(* Logix 5000 Program export KEP; software revision 30.00; part 8 of 15 *)

ADD_ON_INSTRUCTION Ed25519_VERIFY   (* revision 1.0 20170916, vendor Kenneth A. Fischer *)
// Verifies an Ed25519 Signature.
// Revision note:
// Rev1.0: 20170916 - Initial Release
VAR_IN_OUT
   Temp_C1 : DINT[22]; {required}   // Temp C1 value
   Temp_C2 : DINT[22]; {required}   // Temp C2 value
   Temp_C3 : DINT[22]; {required}   // Temp C3 value
   Temp_C4 : DINT[22]; {required}   // Temp C4 value
   Temp_C5 : DINT[22]; {required}   // Temp C5 value
   Temp_C6 : DINT[22]; {required}   // Temp C6 value
   Temp_C7 : DINT[22]; {required}   // Temp C7 value
   Temp_C8 : DINT[22]; {required}   // Temp C8 value
   Temp_C9 : DINT[22]; {required}   // Temp C9 value
   Temp_C10 : DINT[22]; {required}   // Temp C10 value
   Temp_C11 : DINT[22]; {required}   // Temp C11 value
   Temp_C12 : DINT[22]; {required}   // Temp C12 value
   Temp_D1 : DINT[43]; {required}   // Temp D1 value
   Temp_D2 : DINT[43]; {required}   // Temp D2 value
   Temp_E1 : DINT[32]; {required}   // Temp E1 value
   Temp_E2 : DINT[32]; {required}   // Temp E2 value
   Temp_E3 : DINT[32]; {required}   // Temp E3 value
   Temp_L : LINT[4]; {required}   // Temp L value
   Temp_P1 : POINT; {required}
   Temp_P2 : POINT; {required}
   Temp_P3 : POINT; {required}
   Temp_P4 : POINT; {required}
   Temp_MSG : LINT[1600]; {required}   // Temp MSG holder
   Temp_HASH : LINT[8]; {required}   // Temp HASH value
   Inp_Flags : DINT; {required}
   Inp_PubDH : STRING; {required}
   Inp_Ke : STRING; {required}
   Inp_PubKey : STRING; {required}
   Inp_KsID : LINT; {required}
   Inp_KsPrimeID : LINT; {required}
   Inp_Counter : LINT; {required}
   Inp_Sig_R : STRING; {required}
   Inp_Sig_S : STRING; {required}
END_VAR
VAR_OUTPUT
   Out_Status : INT; {access Read Only, visible}
   SEQCTRL_DN : BOOL; {access Read Only}   // Complete
END_VAR
VAR_INPUT
   SEQCTRL_RESET : BOOL;   // Resets Ed25519 Verify if Toggled True
END_VAR
VAR_OUTPUT
   SEQCTRL_STEP : INT; {access Read Only}
   SEQCTRL_SUBSTEP : INT; {access Read Only}
END_VAR
VAR
   SEQCTRL_CMD : DINT;
   SEQCTRL_CMD_TABLE : DINT[70];
   SEQCTRL_DONE : DINT;
   SEQCTRL_NEXT_STEP : INT;
   TEMP : DINT;
   SHA512_SEQ : SHA512_SEQ;
   SEQCTRL_ONS : DINT;
   B512_HtoD : B512_HtoD;
   B256_MODL1 : B256_MODL;
   POINT_MUL1 : POINT_MUL;
   B256_EtoL : B256_EtoL;
   B256_StoC : B256_StoC;
   B256_CtoE : B256_CtoE;
   POINT_DEC1 : POINT_DEC;
   POINT_DEC2 : POINT_DEC;
   POINT_ADD : POINT_ADD;
   B256_StoC_LE : B256_StoC_LE;
   POINT_MUL2 : POINT_MUL;
   EQUAL : BOOL;
   POINT_ENC1 : POINT_ENC;
   POINT_ENC2 : POINT_ENC;
   Wrk_Out : DINT[2];
END_VAR

ROUTINE Logic   (* ladder *)
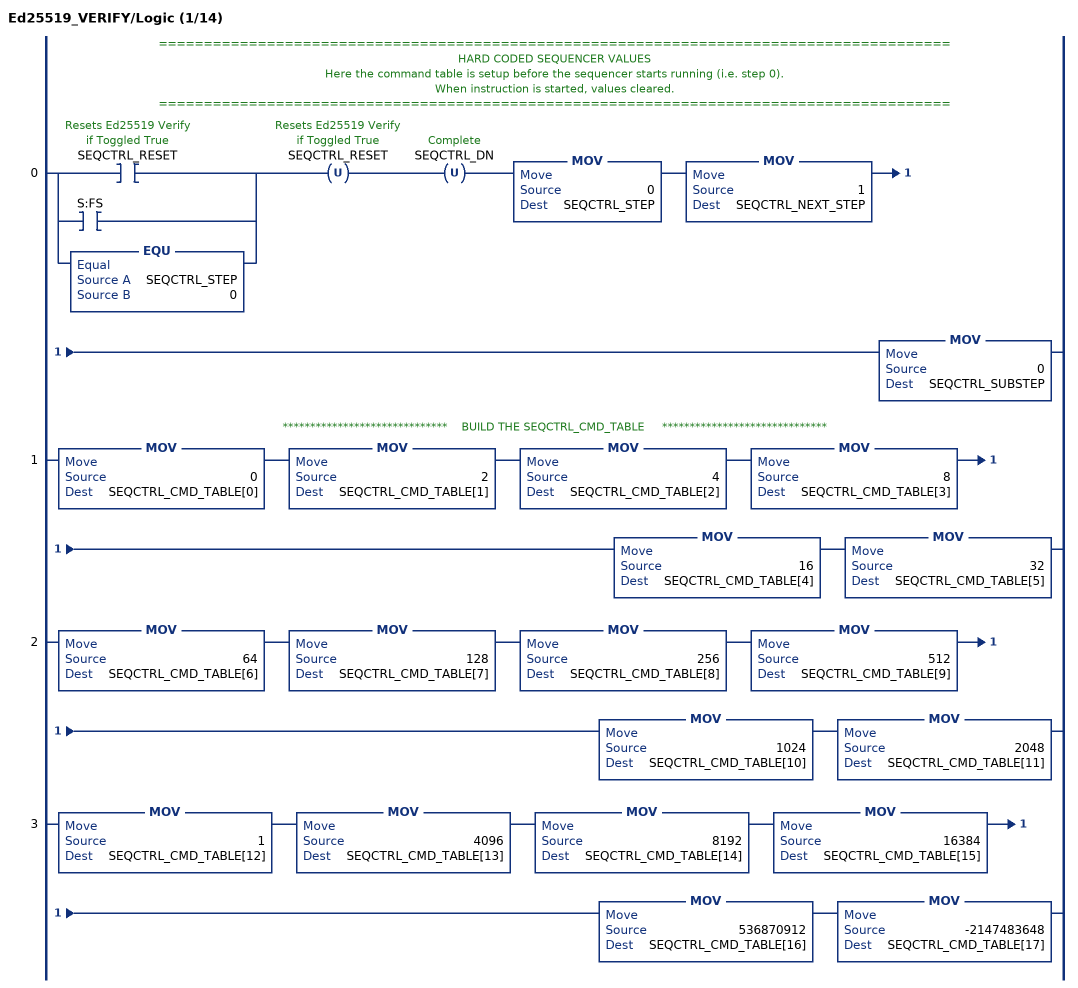
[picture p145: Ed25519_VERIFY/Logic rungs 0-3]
   // ========================================================================================
   // HARD CODED SEQUENCER VALUES
   // Here the command table is setup before the sequencer starts running (i.e. step 0).
   // When instruction is started, values cleared.
   // ========================================================================================
   0: [[XIC(SEQCTRL_RESET) ,XIC(S:FS) ] ,EQU(SEQCTRL_STEP,0) ]OTU(SEQCTRL_RESET)OTU(SEQCTRL_DN)MOV(0,SEQCTRL_STEP)MOV(1,SEQCTRL_NEXT_STEP)MOV(0,SEQCTRL_SUBSTEP);
   // ******************************    BUILD THE SEQCTRL_CMD_TABLE     ******************************
   1: MOV(0,SEQCTRL_CMD_TABLE[0])MOV(2,SEQCTRL_CMD_TABLE[1])MOV(4,SEQCTRL_CMD_TABLE[2])MOV(8,SEQCTRL_CMD_TABLE[3])MOV(16,SEQCTRL_CMD_TABLE[4])MOV(32,SEQCTRL_CMD_TABLE[5]);
   2: MOV(64,SEQCTRL_CMD_TABLE[6])MOV(128,SEQCTRL_CMD_TABLE[7])MOV(256,SEQCTRL_CMD_TABLE[8])MOV(512,SEQCTRL_CMD_TABLE[9])MOV(1024,SEQCTRL_CMD_TABLE[10])MOV(2048,SEQCTRL_CMD_TABLE[11]);
   3: MOV(1,SEQCTRL_CMD_TABLE[12])MOV(4096,SEQCTRL_CMD_TABLE[13])MOV(8192,SEQCTRL_CMD_TABLE[14])MOV(16384,SEQCTRL_CMD_TABLE[15])MOV(536870912,SEQCTRL_CMD_TABLE[16])MOV(-2147483648,SEQCTRL_CMD_TABLE[17]);
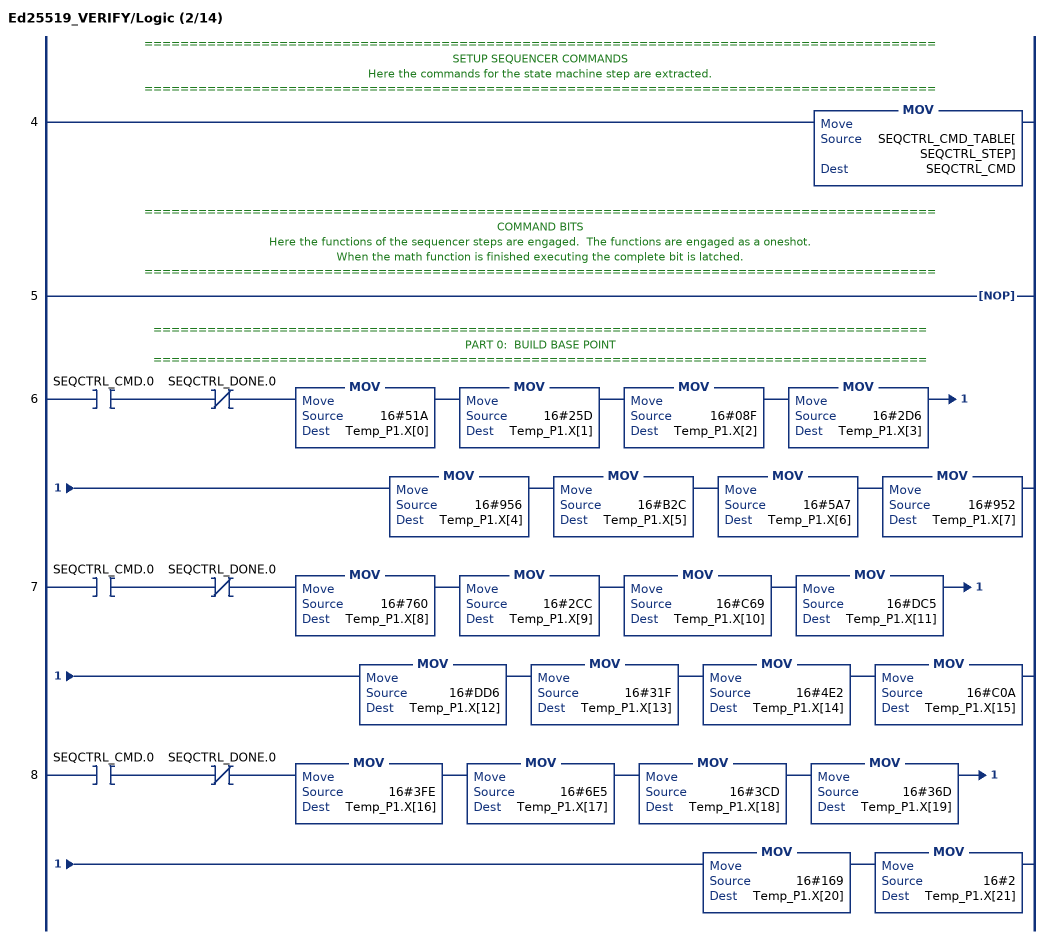
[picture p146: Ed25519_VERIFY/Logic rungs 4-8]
   // ========================================================================================
   // SETUP SEQUENCER COMMANDS
   // Here the commands for the state machine step are extracted.
   // ========================================================================================
   4: MOV(SEQCTRL_CMD_TABLE[SEQCTRL_STEP],SEQCTRL_CMD);
   // ========================================================================================
   // COMMAND BITS
   // Here the functions of the sequencer steps are engaged.  The functions are engaged as a oneshot.
   // When the math function is finished executing the complete bit is latched.
   // ========================================================================================
   5: NOP();
   // ======================================================================================
   // PART 0:  BUILD BASE POINT
   // ======================================================================================
   6: XIC(SEQCTRL_CMD.0)XIO(SEQCTRL_DONE.0)MOV(16#51A,Temp_P1.X[0])MOV(16#25D,Temp_P1.X[1])MOV(16#08F,Temp_P1.X[2])MOV(16#2D6,Temp_P1.X[3])MOV(16#956,Temp_P1.X[4])MOV(16#B2C,Temp_P1.X[5])MOV(16#5A7,Temp_P1.X[6])MOV(16#952,Temp_P1.X[7]);
   7: XIC(SEQCTRL_CMD.0)XIO(SEQCTRL_DONE.0)MOV(16#760,Temp_P1.X[8])MOV(16#2CC,Temp_P1.X[9])MOV(16#C69,Temp_P1.X[10])MOV(16#DC5,Temp_P1.X[11])MOV(16#DD6,Temp_P1.X[12])MOV(16#31F,Temp_P1.X[13])MOV(16#4E2,Temp_P1.X[14])MOV(16#C0A,Temp_P1.X[15]);
   8: XIC(SEQCTRL_CMD.0)XIO(SEQCTRL_DONE.0)MOV(16#3FE,Temp_P1.X[16])MOV(16#6E5,Temp_P1.X[17])MOV(16#3CD,Temp_P1.X[18])MOV(16#36D,Temp_P1.X[19])MOV(16#169,Temp_P1.X[20])MOV(16#2,Temp_P1.X[21]);
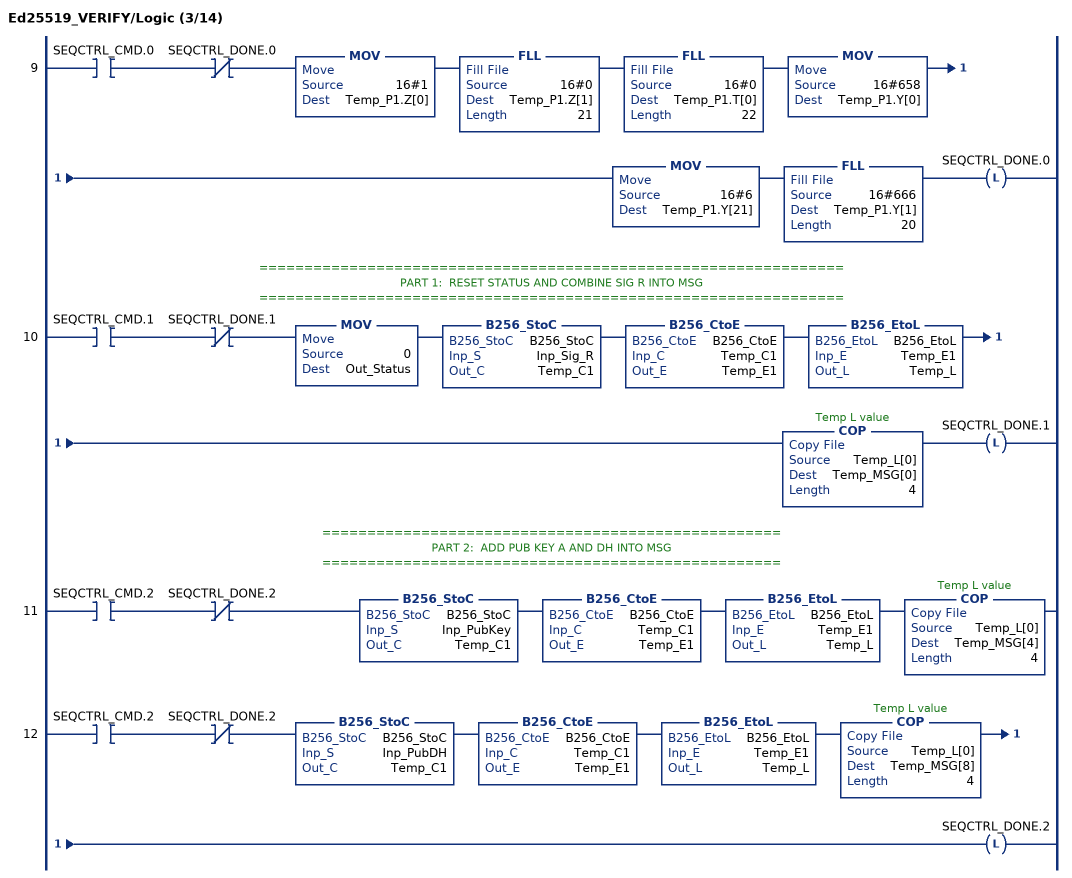
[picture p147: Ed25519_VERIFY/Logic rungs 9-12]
   9: XIC(SEQCTRL_CMD.0)XIO(SEQCTRL_DONE.0)MOV(16#1,Temp_P1.Z[0])FLL(16#0,Temp_P1.Z[1],21)FLL(16#0,Temp_P1.T[0],22)MOV(16#658,Temp_P1.Y[0])MOV(16#6,Temp_P1.Y[21])FLL(16#666,Temp_P1.Y[1],20)OTL(SEQCTRL_DONE.0);
   // =================================================================
   // PART 1:  RESET STATUS AND COMBINE SIG R INTO MSG
   // =================================================================
   10: XIC(SEQCTRL_CMD.1)XIO(SEQCTRL_DONE.1)MOV(0,Out_Status)B256_StoC(B256_StoC,Inp_Sig_R,Temp_C1)B256_CtoE(B256_CtoE,Temp_C1,Temp_E1)B256_EtoL(B256_EtoL,Temp_E1,Temp_L)COP(Temp_L[0],Temp_MSG[0],4)OTL(SEQCTRL_DONE.1);
   // ===================================================
   // PART 2:  ADD PUB KEY A AND DH INTO MSG
   // ===================================================
   11: XIC(SEQCTRL_CMD.2)XIO(SEQCTRL_DONE.2)B256_StoC(B256_StoC,Inp_PubKey,Temp_C1)B256_CtoE(B256_CtoE,Temp_C1,Temp_E1)B256_EtoL(B256_EtoL,Temp_E1,Temp_L)COP(Temp_L[0],Temp_MSG[4],4);
   12: XIC(SEQCTRL_CMD.2)XIO(SEQCTRL_DONE.2)B256_StoC(B256_StoC,Inp_PubDH,Temp_C1)B256_CtoE(B256_CtoE,Temp_C1,Temp_E1)B256_EtoL(B256_EtoL,Temp_E1,Temp_L)COP(Temp_L[0],Temp_MSG[8],4)OTL(SEQCTRL_DONE.2);
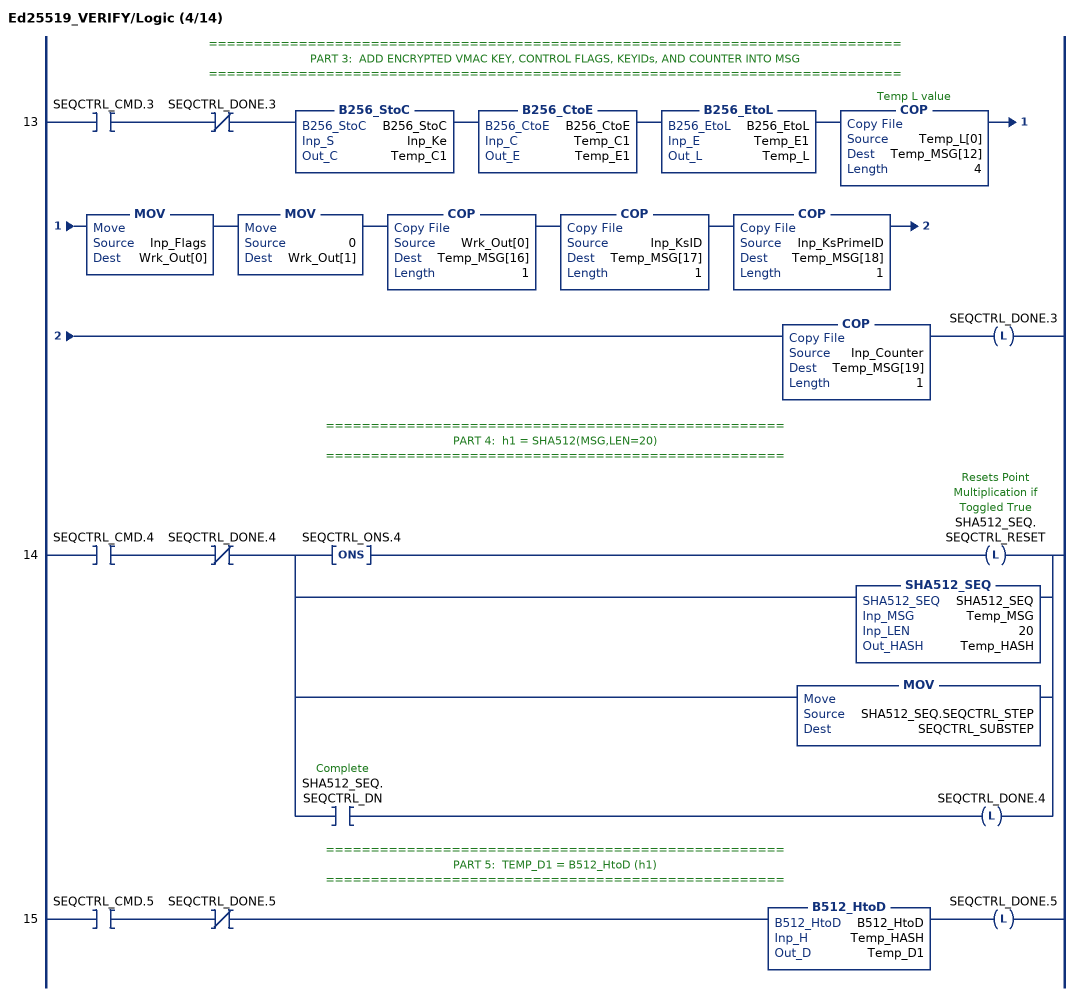
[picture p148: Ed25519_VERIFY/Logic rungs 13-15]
   // =============================================================================
   // PART 3:  ADD ENCRYPTED VMAC KEY, CONTROL FLAGS, KEYIDs, AND COUNTER INTO MSG
   // =============================================================================
   13: XIC(SEQCTRL_CMD.3)XIO(SEQCTRL_DONE.3)B256_StoC(B256_StoC,Inp_Ke,Temp_C1)B256_CtoE(B256_CtoE,Temp_C1,Temp_E1)B256_EtoL(B256_EtoL,Temp_E1,Temp_L)COP(Temp_L[0],Temp_MSG[12],4)MOV(Inp_Flags,Wrk_Out[0])MOV(0,Wrk_Out[1])COP(Wrk_Out[0],Temp_MSG[16],1)COP(Inp_KsID,Temp_MSG[17],1)COP(Inp_KsPrimeID,Temp_MSG[18],1)COP(Inp_Counter,Temp_MSG[19],1)OTL(SEQCTRL_DONE.3);
   // ===================================================
   // PART 4:  h1 = SHA512(MSG,LEN=20)
   // ===================================================
   14: XIC(SEQCTRL_CMD.4)XIO(SEQCTRL_DONE.4)[ONS(SEQCTRL_ONS.4) OTL(SHA512_SEQ.SEQCTRL_RESET) ,SHA512_SEQ(SHA512_SEQ,Temp_MSG,20,Temp_HASH) ,MOV(SHA512_SEQ.SEQCTRL_STEP,SEQCTRL_SUBSTEP) ,XIC(SHA512_SEQ.SEQCTRL_DN) OTL(SEQCTRL_DONE.4) ];
   // ===================================================
   // PART 5:  TEMP_D1 = B512_HtoD (h1)
   // ===================================================
   15: XIC(SEQCTRL_CMD.5)XIO(SEQCTRL_DONE.5)B512_HtoD(B512_HtoD,Temp_HASH,Temp_D1)OTL(SEQCTRL_DONE.5);
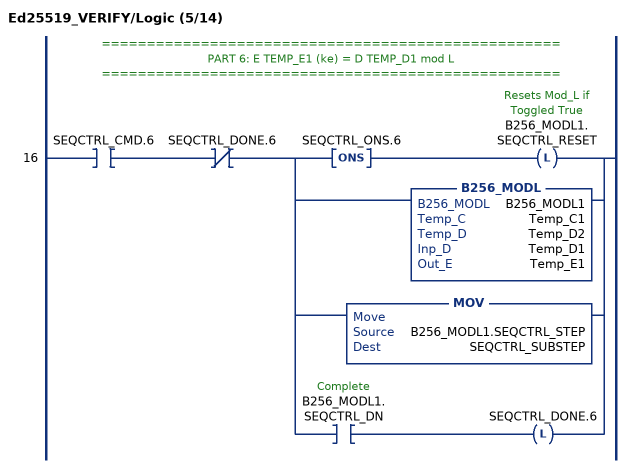
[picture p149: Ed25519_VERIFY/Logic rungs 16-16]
   // ===================================================
   // PART 6: E TEMP_E1 (ke) = D TEMP_D1 mod L
   // ===================================================
   16: XIC(SEQCTRL_CMD.6)XIO(SEQCTRL_DONE.6)[ONS(SEQCTRL_ONS.6) OTL(B256_MODL1.SEQCTRL_RESET) ,B256_MODL(B256_MODL1,Temp_C1,Temp_D2,Temp_D1,Temp_E1) ,MOV(B256_MODL1.SEQCTRL_STEP,SEQCTRL_SUBSTEP) ,XIC(B256_MODL1.SEQCTRL_DN) OTL(SEQCTRL_DONE.6) ];
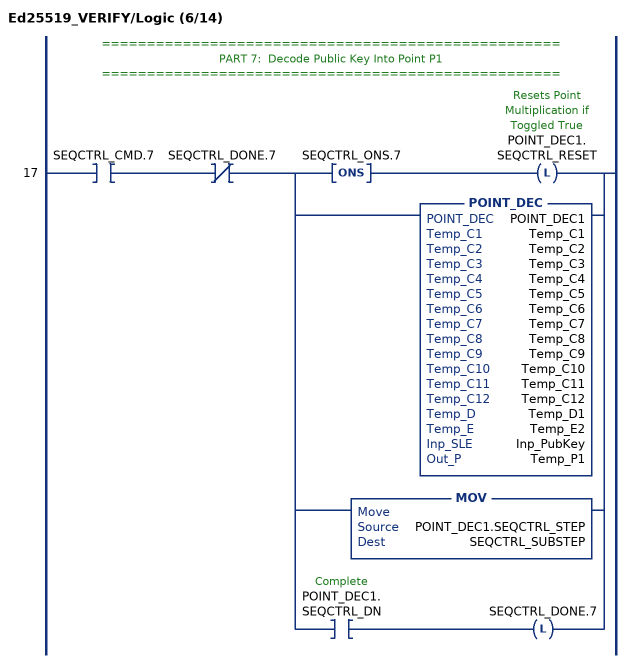
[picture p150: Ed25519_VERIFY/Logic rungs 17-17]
   // ===================================================
   // PART 7:  Decode Public Key Into Point P1
   // ===================================================
   17: XIC(SEQCTRL_CMD.7)XIO(SEQCTRL_DONE.7)[ONS(SEQCTRL_ONS.7) OTL(POINT_DEC1.SEQCTRL_RESET) ,POINT_DEC(POINT_DEC1,Temp_C1,Temp_C2,Temp_C3,Temp_C4,Temp_C5,Temp_C6,Temp_C7,Temp_C8,Temp_C9,Temp_C10,Temp_C11,Temp_C12,Temp_D1,Temp_E2,Inp_PubKey,Temp_P1) ,MOV(POINT_DEC1.SEQCTRL_STEP,SEQCTRL_SUBSTEP) ,XIC(POINT_DEC1.SEQCTRL_DN) OTL(SEQCTRL_DONE.7) ];
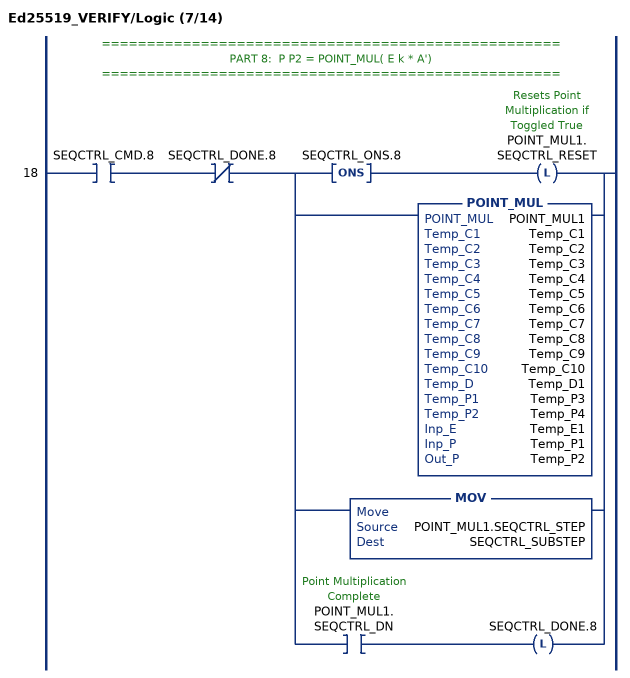
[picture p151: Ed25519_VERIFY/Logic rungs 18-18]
   // ===================================================
   // PART 8:  P P2 = POINT_MUL( E k * A')
   // ===================================================
   18: XIC(SEQCTRL_CMD.8)XIO(SEQCTRL_DONE.8)[ONS(SEQCTRL_ONS.8) OTL(POINT_MUL1.SEQCTRL_RESET) ,POINT_MUL(POINT_MUL1,Temp_C1,Temp_C2,Temp_C3,Temp_C4,Temp_C5,Temp_C6,Temp_C7,Temp_C8,Temp_C9,Temp_C10,Temp_D1,Temp_P3,Temp_P4,Temp_E1,Temp_P1,Temp_P2) ,MOV(POINT_MUL1.SEQCTRL_STEP,SEQCTRL_SUBSTEP) ,XIC(POINT_MUL1.SEQCTRL_DN) OTL(SEQCTRL_DONE.8) ];
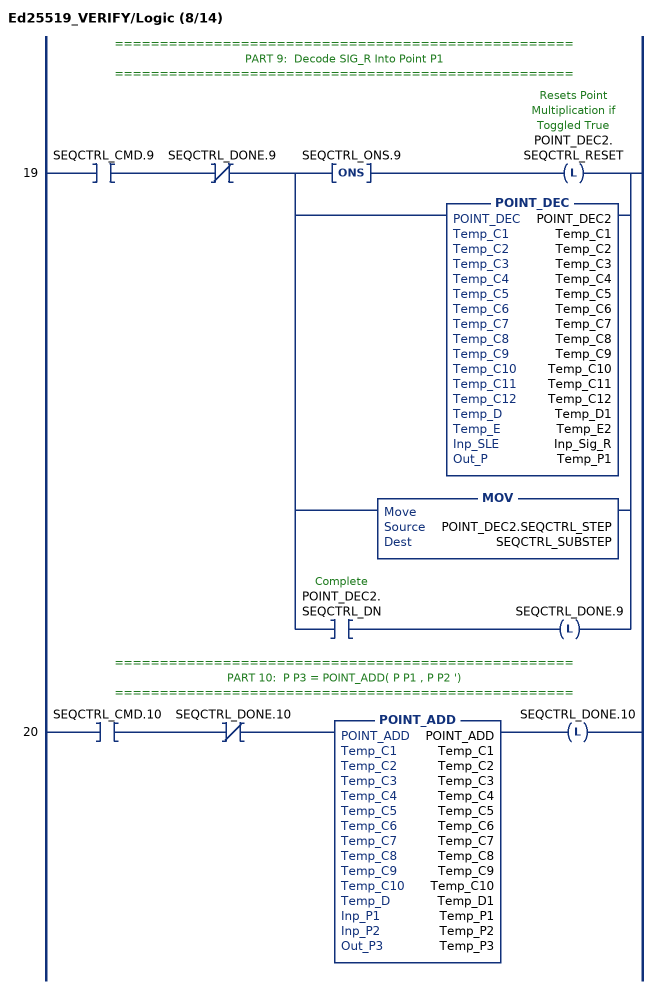
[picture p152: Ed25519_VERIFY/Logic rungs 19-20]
   // ===================================================
   // PART 9:  Decode SIG_R Into Point P1
   // ===================================================
   19: XIC(SEQCTRL_CMD.9)XIO(SEQCTRL_DONE.9)[ONS(SEQCTRL_ONS.9) OTL(POINT_DEC2.SEQCTRL_RESET) ,POINT_DEC(POINT_DEC2,Temp_C1,Temp_C2,Temp_C3,Temp_C4,Temp_C5,Temp_C6,Temp_C7,Temp_C8,Temp_C9,Temp_C10,Temp_C11,Temp_C12,Temp_D1,Temp_E2,Inp_Sig_R,Temp_P1) ,MOV(POINT_DEC2.SEQCTRL_STEP,SEQCTRL_SUBSTEP) ,XIC(POINT_DEC2.SEQCTRL_DN) OTL(SEQCTRL_DONE.9) ];
   // ===================================================
   // PART 10:  P P3 = POINT_ADD( P P1 , P P2 ')
   // ===================================================
   20: XIC(SEQCTRL_CMD.10)XIO(SEQCTRL_DONE.10)POINT_ADD(POINT_ADD,Temp_C1,Temp_C2,Temp_C3,Temp_C4,Temp_C5,Temp_C6,Temp_C7,Temp_C8,Temp_C9,Temp_C10,Temp_D1,Temp_P1,Temp_P2,Temp_P3)OTL(SEQCTRL_DONE.10);
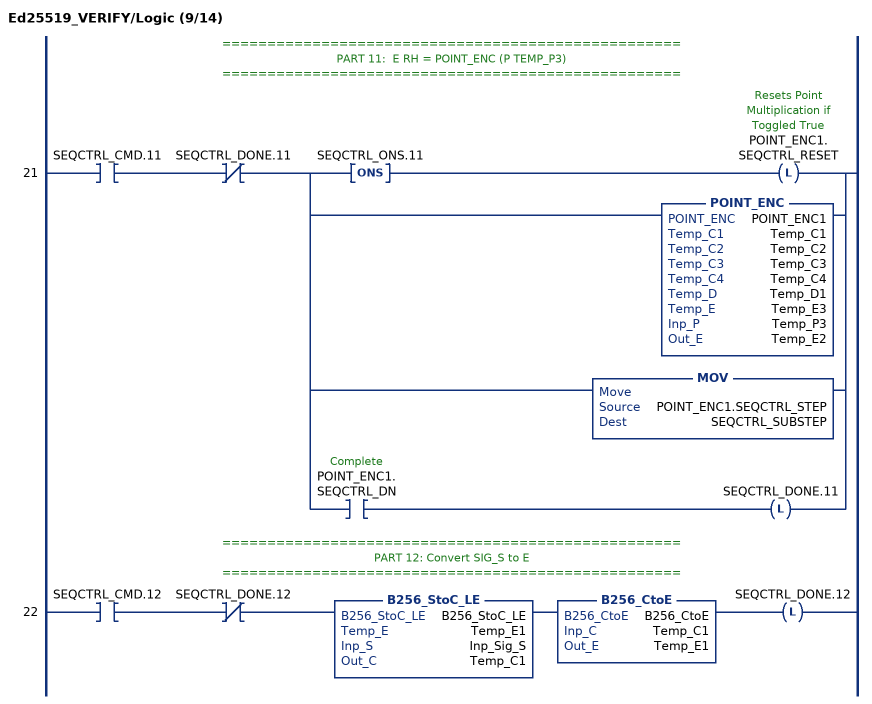
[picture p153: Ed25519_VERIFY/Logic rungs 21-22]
   // ===================================================
   // PART 11:  E RH = POINT_ENC (P TEMP_P3)
   // ===================================================
   21: XIC(SEQCTRL_CMD.11)XIO(SEQCTRL_DONE.11)[ONS(SEQCTRL_ONS.11) OTL(POINT_ENC1.SEQCTRL_RESET) ,POINT_ENC(POINT_ENC1,Temp_C1,Temp_C2,Temp_C3,Temp_C4,Temp_D1,Temp_E3,Temp_P3,Temp_E2) ,MOV(POINT_ENC1.SEQCTRL_STEP,SEQCTRL_SUBSTEP) ,XIC(POINT_ENC1.SEQCTRL_DN) OTL(SEQCTRL_DONE.11) ];
   // ===================================================
   // PART 12: Convert SIG_S to E
   // ===================================================
   22: XIC(SEQCTRL_CMD.12)XIO(SEQCTRL_DONE.12)B256_StoC_LE(B256_StoC_LE,Temp_E1,Inp_Sig_S,Temp_C1)B256_CtoE(B256_CtoE,Temp_C1,Temp_E1)OTL(SEQCTRL_DONE.12);
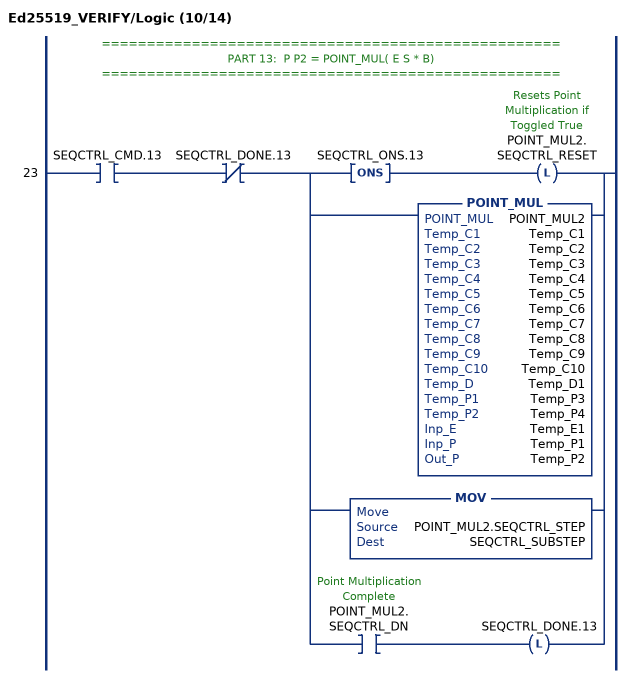
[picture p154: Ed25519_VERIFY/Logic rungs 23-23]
   // ===================================================
   // PART 13:  P P2 = POINT_MUL( E S * B)
   // ===================================================
   23: XIC(SEQCTRL_CMD.13)XIO(SEQCTRL_DONE.13)[ONS(SEQCTRL_ONS.13) OTL(POINT_MUL2.SEQCTRL_RESET) ,POINT_MUL(POINT_MUL2,Temp_C1,Temp_C2,Temp_C3,Temp_C4,Temp_C5,Temp_C6,Temp_C7,Temp_C8,Temp_C9,Temp_C10,Temp_D1,Temp_P3,Temp_P4,Temp_E1,Temp_P1,Temp_P2) ,MOV(POINT_MUL2.SEQCTRL_STEP,SEQCTRL_SUBSTEP) ,XIC(POINT_MUL2.SEQCTRL_DN) OTL(SEQCTRL_DONE.13) ];
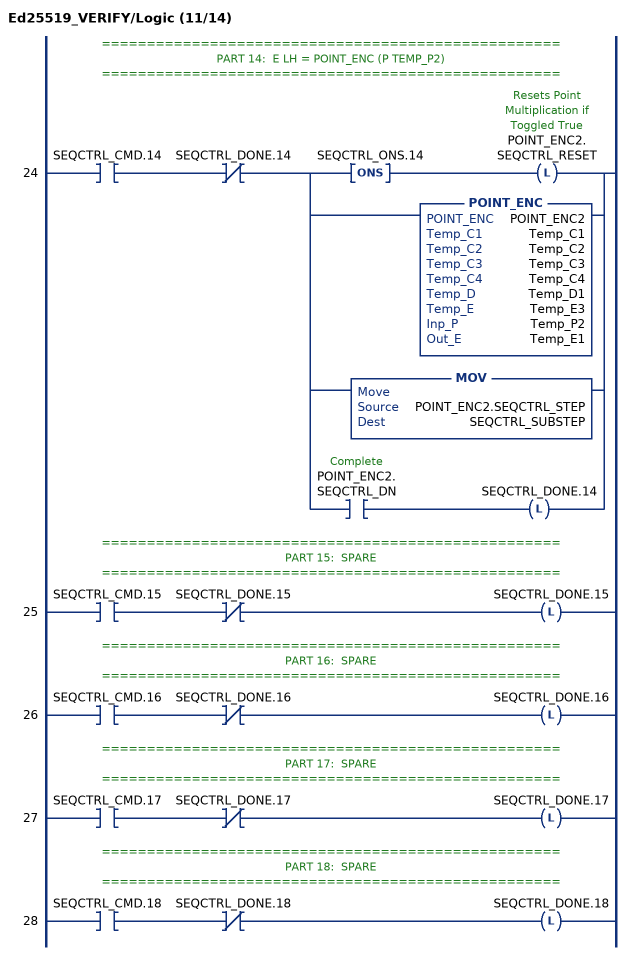
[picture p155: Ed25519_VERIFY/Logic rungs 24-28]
   // ===================================================
   // PART 14:  E LH = POINT_ENC (P TEMP_P2)
   // ===================================================
   24: XIC(SEQCTRL_CMD.14)XIO(SEQCTRL_DONE.14)[ONS(SEQCTRL_ONS.14) OTL(POINT_ENC2.SEQCTRL_RESET) ,POINT_ENC(POINT_ENC2,Temp_C1,Temp_C2,Temp_C3,Temp_C4,Temp_D1,Temp_E3,Temp_P2,Temp_E1) ,MOV(POINT_ENC2.SEQCTRL_STEP,SEQCTRL_SUBSTEP) ,XIC(POINT_ENC2.SEQCTRL_DN) OTL(SEQCTRL_DONE.14) ];
   // ===================================================
   // PART 15:  SPARE
   // ===================================================
   25: XIC(SEQCTRL_CMD.15)XIO(SEQCTRL_DONE.15)OTL(SEQCTRL_DONE.15);
   // ===================================================
   // PART 16:  SPARE
   // ===================================================
   26: XIC(SEQCTRL_CMD.16)XIO(SEQCTRL_DONE.16)OTL(SEQCTRL_DONE.16);
   // ===================================================
   // PART 17:  SPARE
   // ===================================================
   27: XIC(SEQCTRL_CMD.17)XIO(SEQCTRL_DONE.17)OTL(SEQCTRL_DONE.17);
   // ===================================================
   // PART 18:  SPARE
   // ===================================================
   28: XIC(SEQCTRL_CMD.18)XIO(SEQCTRL_DONE.18)OTL(SEQCTRL_DONE.18);
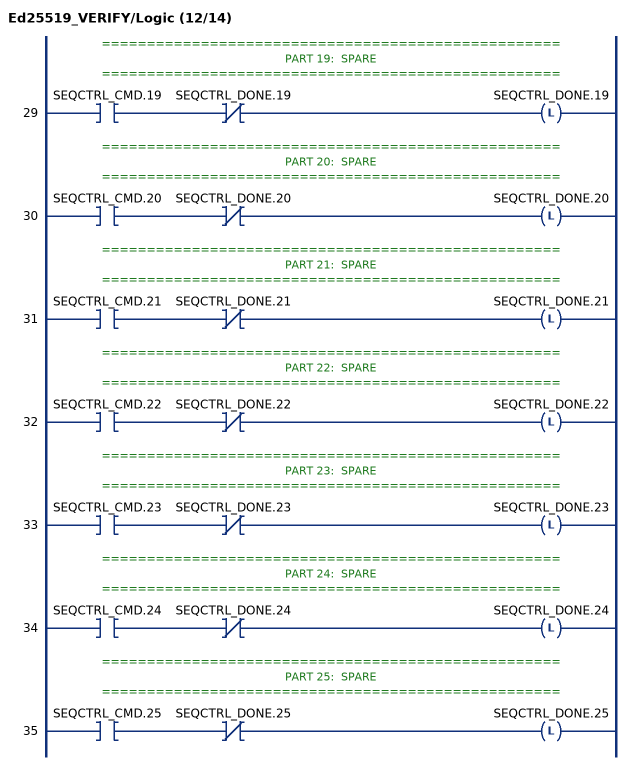
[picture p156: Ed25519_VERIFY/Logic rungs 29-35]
   // ===================================================
   // PART 19:  SPARE
   // ===================================================
   29: XIC(SEQCTRL_CMD.19)XIO(SEQCTRL_DONE.19)OTL(SEQCTRL_DONE.19);
   // ===================================================
   // PART 20:  SPARE
   // ===================================================
   30: XIC(SEQCTRL_CMD.20)XIO(SEQCTRL_DONE.20)OTL(SEQCTRL_DONE.20);
   // ===================================================
   // PART 21:  SPARE
   // ===================================================
   31: XIC(SEQCTRL_CMD.21)XIO(SEQCTRL_DONE.21)OTL(SEQCTRL_DONE.21);
   // ===================================================
   // PART 22:  SPARE
   // ===================================================
   32: XIC(SEQCTRL_CMD.22)XIO(SEQCTRL_DONE.22)OTL(SEQCTRL_DONE.22);
   // ===================================================
   // PART 23:  SPARE
   // ===================================================
   33: XIC(SEQCTRL_CMD.23)XIO(SEQCTRL_DONE.23)OTL(SEQCTRL_DONE.23);
   // ===================================================
   // PART 24:  SPARE
   // ===================================================
   34: XIC(SEQCTRL_CMD.24)XIO(SEQCTRL_DONE.24)OTL(SEQCTRL_DONE.24);
   // ===================================================
   // PART 25:  SPARE
   // ===================================================
   35: XIC(SEQCTRL_CMD.25)XIO(SEQCTRL_DONE.25)OTL(SEQCTRL_DONE.25);
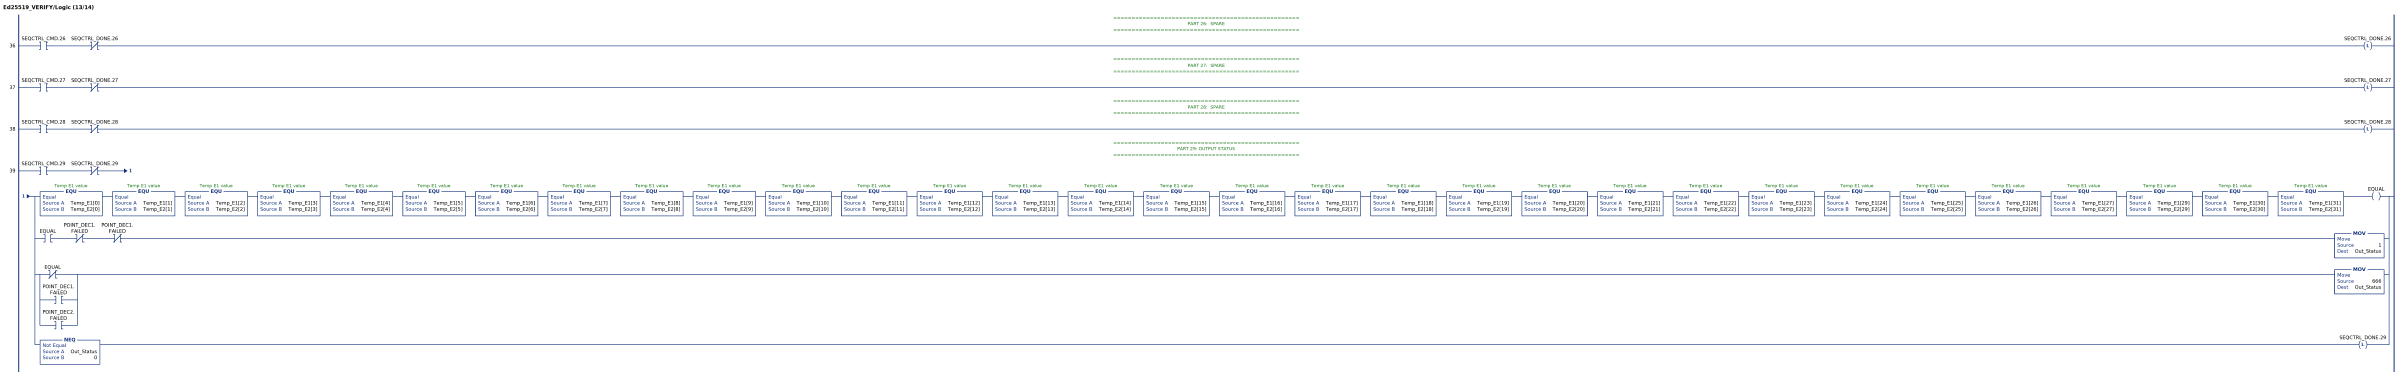
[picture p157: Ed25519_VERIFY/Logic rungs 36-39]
   // ===================================================
   // PART 26:  SPARE
   // ===================================================
   36: XIC(SEQCTRL_CMD.26)XIO(SEQCTRL_DONE.26)OTL(SEQCTRL_DONE.26);
   // ===================================================
   // PART 27:  SPARE
   // ===================================================
   37: XIC(SEQCTRL_CMD.27)XIO(SEQCTRL_DONE.27)OTL(SEQCTRL_DONE.27);
   // ===================================================
   // PART 28:  SPARE
   // ===================================================
   38: XIC(SEQCTRL_CMD.28)XIO(SEQCTRL_DONE.28)OTL(SEQCTRL_DONE.28);
   // ===================================================
   // PART 29: OUTPUT STATUS
   // ===================================================
   39: XIC(SEQCTRL_CMD.29)XIO(SEQCTRL_DONE.29)[EQU(Temp_E1[0],Temp_E2[0]) EQU(Temp_E1[1],Temp_E2[1]) EQU(Temp_E1[2],Temp_E2[2]) EQU(Temp_E1[3],Temp_E2[3]) EQU(Temp_E1[4],Temp_E2[4]) EQU(Temp_E1[5],Temp_E2[5]) EQU(Temp_E1[6],Temp_E2[6]) EQU(Temp_E1[7],Temp_E2[7]) EQU(Temp_E1[8],Temp_E2[8]) EQU(Temp_E1[9],Temp_E2[9]) EQU(Temp_E1[10],Temp_E2[10]) EQU(Temp_E1[11],Temp_E2[11]) EQU(Temp_E1[12],Temp_E2[12]) EQU(Temp_E1[13],Temp_E2[13]) EQU(Temp_E1[14],Temp_E2[14]) EQU(Temp_E1[15],Temp_E2[15]) EQU(Temp_E1[16],Temp_E2[16]) EQU(Temp_E1[17],Temp_E2[17]) EQU(Temp_E1[18],Temp_E2[18]) EQU(Temp_E1[19],Temp_E2[19]) EQU(Temp_E1[20],Temp_E2[20]) EQU(Temp_E1[21],Temp_E2[21]) EQU(Temp_E1[22],Temp_E2[22]) EQU(Temp_E1[23],Temp_E2[23]) EQU(Temp_E1[24],Temp_E2[24]) EQU(Temp_E1[25],Temp_E2[25]) EQU(Temp_E1[26],Temp_E2[26]) EQU(Temp_E1[27],Temp_E2[27]) EQU(Temp_E1[29],Temp_E2[29]) EQU(Temp_E1[30],Temp_E2[30]) EQU(Temp_E1[31],Temp_E2[31]) OTE(EQUAL) ,XIC(EQUAL) XIO(POINT_DEC1.FAILED) XIO(POINT_DEC1.FAILED) MOV(1,Out_Status) ,[XIO(EQUAL) ,XIC(POINT_DEC1.FAILED) ,XIC(POINT_DEC2.FAILED) ] MOV(666,Out_Status) ,NEQ(Out_Status,0) OTL(SEQCTRL_DONE.29) ];
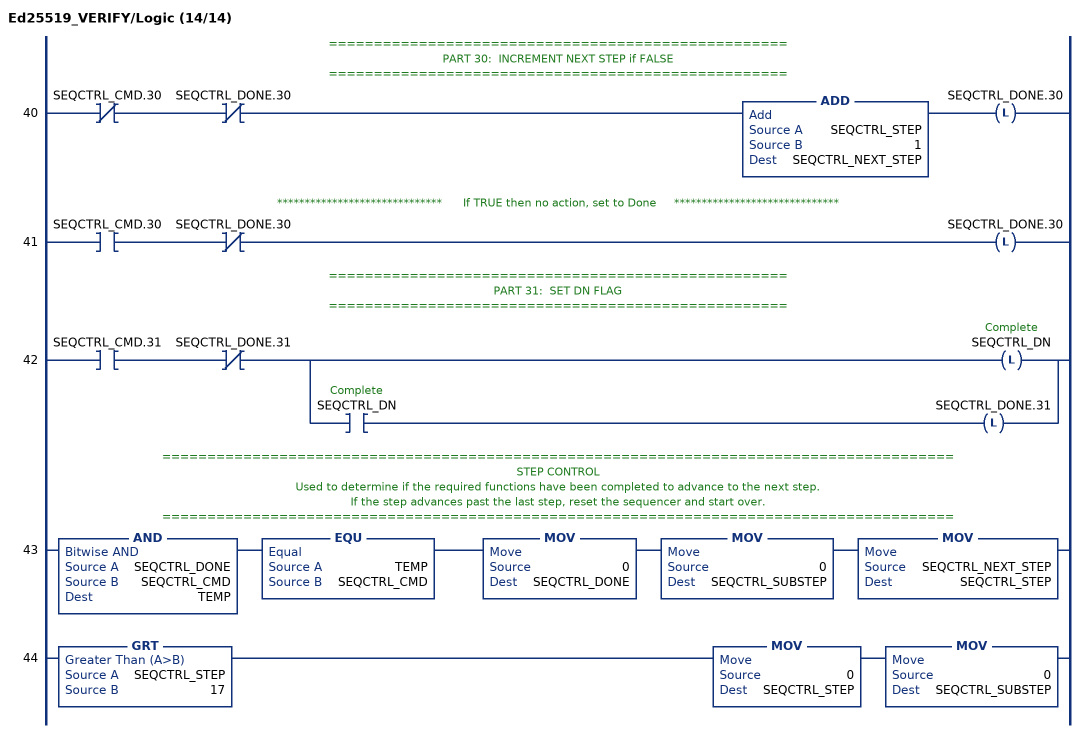
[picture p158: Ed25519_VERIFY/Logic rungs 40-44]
   // ===================================================
   // PART 30:  INCREMENT NEXT STEP if FALSE
   // ===================================================
   40: XIO(SEQCTRL_CMD.30)XIO(SEQCTRL_DONE.30)ADD(SEQCTRL_STEP,1,SEQCTRL_NEXT_STEP)OTL(SEQCTRL_DONE.30);
   // ******************************      If TRUE then no action, set to Done     ******************************
   41: XIC(SEQCTRL_CMD.30)XIO(SEQCTRL_DONE.30)OTL(SEQCTRL_DONE.30);
   // ===================================================
   // PART 31:  SET DN FLAG
   // ===================================================
   42: XIC(SEQCTRL_CMD.31)XIO(SEQCTRL_DONE.31)[OTL(SEQCTRL_DN) ,XIC(SEQCTRL_DN) OTL(SEQCTRL_DONE.31) ];
   // ========================================================================================
   // STEP CONTROL
   // Used to determine if the required functions have been completed to advance to the next step.
   // If the step advances past the last step, reset the sequencer and start over.
   // ========================================================================================
   43: AND(SEQCTRL_DONE,SEQCTRL_CMD,TEMP)EQU(TEMP,SEQCTRL_CMD)MOV(0,SEQCTRL_DONE)MOV(0,SEQCTRL_SUBSTEP)MOV(SEQCTRL_NEXT_STEP,SEQCTRL_STEP);
   44: GRT(SEQCTRL_STEP,17)MOV(0,SEQCTRL_STEP)MOV(0,SEQCTRL_SUBSTEP);
END_ROUTINE
END_ADD_ON_INSTRUCTION

ADD_ON_INSTRUCTION PRNG   (* revision 1.0 20170916, vendor Kenneth A. Fischer *)
// Pseudo-Random Number Generator
// (not proven secure)
// Revision note:
// Rev1.0: 20170916 - Initial Release
VAR_IN_OUT
   Temp_C : DINT[22]; {required}
   Temp_D : DINT[43]; {required}
   Temp_E : DINT[32]; {required}
   Temp_L : LINT[4]; {required}
   Temp_MSG : LINT[1600]; {required}   // Temp MSG holder
   Temp_HASH : LINT[8]; {required}   // Temp HASH value
   Inp_Constant : STRING; {required}
   Inp_Seed : LINT[13]; {required}
   Inp_Counter : LINT; {required}
   Out_PRN : STRING; {required}
END_VAR
VAR_OUTPUT
   SEQCTRL_DN : BOOL; {access Read Only}   // Complete
END_VAR
VAR_INPUT
   SEQCTRL_RESET : BOOL;   // Resets Ed25519 Verify if Toggled True
END_VAR
VAR_OUTPUT
   SEQCTRL_STEP : INT; {access Read Only}
   SEQCTRL_SUBSTEP : INT; {access Read Only}
END_VAR
VAR
   SEQCTRL_CMD : DINT;
   SEQCTRL_CMD_TABLE : DINT[70];
   SEQCTRL_DONE : DINT;
   SEQCTRL_NEXT_STEP : INT;
   TEMP : DINT;
   SHA512_SEQ : SHA512_SEQ;
   SEQCTRL_ONS : DINT;
   Wrk_Out : DINT[2];
   L_INC : L_INC;
   B256_StoC : B256_StoC;
   B256_CtoE : B256_CtoE;
   B256_EtoL : B256_EtoL;
   B512_HtoD : B512_HtoD;
   B256_CtoS : B256_CtoS;
   L_ROTR : L_ROTR;
   L_ADD : L_ADD;
   SwapLint : LINT;
END_VAR

ROUTINE Logic   (* ladder *)
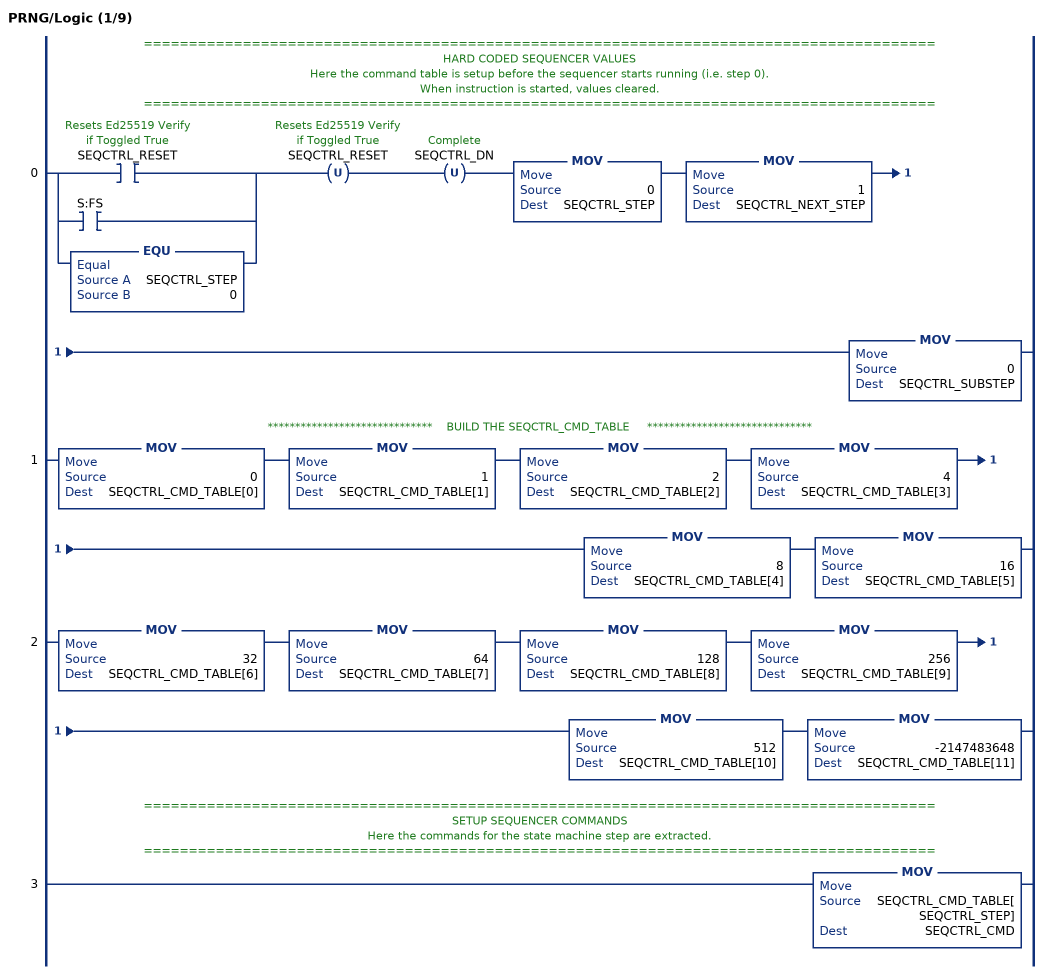
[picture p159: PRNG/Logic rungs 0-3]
   // ========================================================================================
   // HARD CODED SEQUENCER VALUES
   // Here the command table is setup before the sequencer starts running (i.e. step 0).
   // When instruction is started, values cleared.
   // ========================================================================================
   0: [[XIC(SEQCTRL_RESET) ,XIC(S:FS) ] ,EQU(SEQCTRL_STEP,0) ]OTU(SEQCTRL_RESET)OTU(SEQCTRL_DN)MOV(0,SEQCTRL_STEP)MOV(1,SEQCTRL_NEXT_STEP)MOV(0,SEQCTRL_SUBSTEP);
   // ******************************    BUILD THE SEQCTRL_CMD_TABLE     ******************************
   1: MOV(0,SEQCTRL_CMD_TABLE[0])MOV(1,SEQCTRL_CMD_TABLE[1])MOV(2,SEQCTRL_CMD_TABLE[2])MOV(4,SEQCTRL_CMD_TABLE[3])MOV(8,SEQCTRL_CMD_TABLE[4])MOV(16,SEQCTRL_CMD_TABLE[5]);
   2: MOV(32,SEQCTRL_CMD_TABLE[6])MOV(64,SEQCTRL_CMD_TABLE[7])MOV(128,SEQCTRL_CMD_TABLE[8])MOV(256,SEQCTRL_CMD_TABLE[9])MOV(512,SEQCTRL_CMD_TABLE[10])MOV(-2147483648,SEQCTRL_CMD_TABLE[11]);
   // ========================================================================================
   // SETUP SEQUENCER COMMANDS
   // Here the commands for the state machine step are extracted.
   // ========================================================================================
   3: MOV(SEQCTRL_CMD_TABLE[SEQCTRL_STEP],SEQCTRL_CMD);
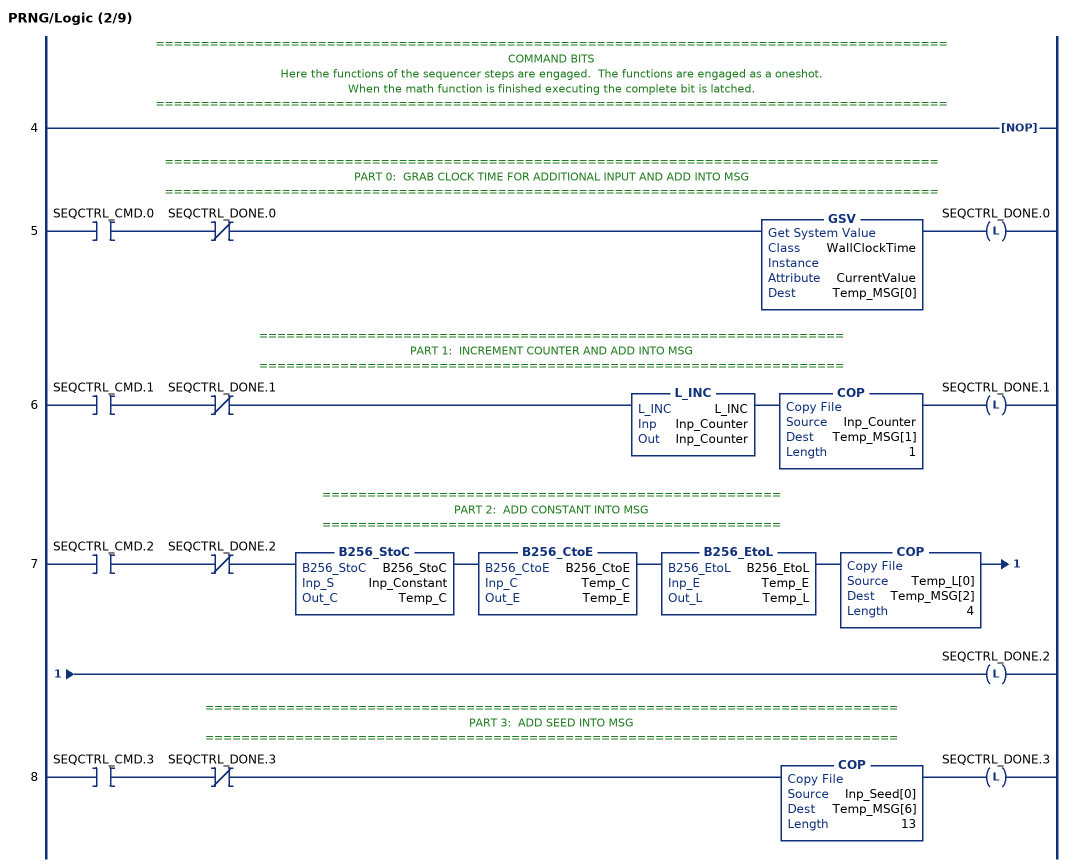
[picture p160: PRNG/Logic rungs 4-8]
   // ========================================================================================
   // COMMAND BITS
   // Here the functions of the sequencer steps are engaged.  The functions are engaged as a oneshot.
   // When the math function is finished executing the complete bit is latched.
   // ========================================================================================
   4: NOP();
   // ======================================================================================
   // PART 0:  GRAB CLOCK TIME FOR ADDITIONAL INPUT AND ADD INTO MSG
   // ======================================================================================
   5: XIC(SEQCTRL_CMD.0)XIO(SEQCTRL_DONE.0)GSV(WallClockTime,,CurrentValue,Temp_MSG[0])OTL(SEQCTRL_DONE.0);
   // =================================================================
   // PART 1:  INCREMENT COUNTER AND ADD INTO MSG
   // =================================================================
   6: XIC(SEQCTRL_CMD.1)XIO(SEQCTRL_DONE.1)L_INC(L_INC,Inp_Counter,Inp_Counter)COP(Inp_Counter,Temp_MSG[1],1)OTL(SEQCTRL_DONE.1);
   // ===================================================
   // PART 2:  ADD CONSTANT INTO MSG
   // ===================================================
   7: XIC(SEQCTRL_CMD.2)XIO(SEQCTRL_DONE.2)B256_StoC(B256_StoC,Inp_Constant,Temp_C)B256_CtoE(B256_CtoE,Temp_C,Temp_E)B256_EtoL(B256_EtoL,Temp_E,Temp_L)COP(Temp_L[0],Temp_MSG[2],4)OTL(SEQCTRL_DONE.2);
   // =============================================================================
   // PART 3:  ADD SEED INTO MSG
   // =============================================================================
   8: XIC(SEQCTRL_CMD.3)XIO(SEQCTRL_DONE.3)COP(Inp_Seed[0],Temp_MSG[6],13)OTL(SEQCTRL_DONE.3);
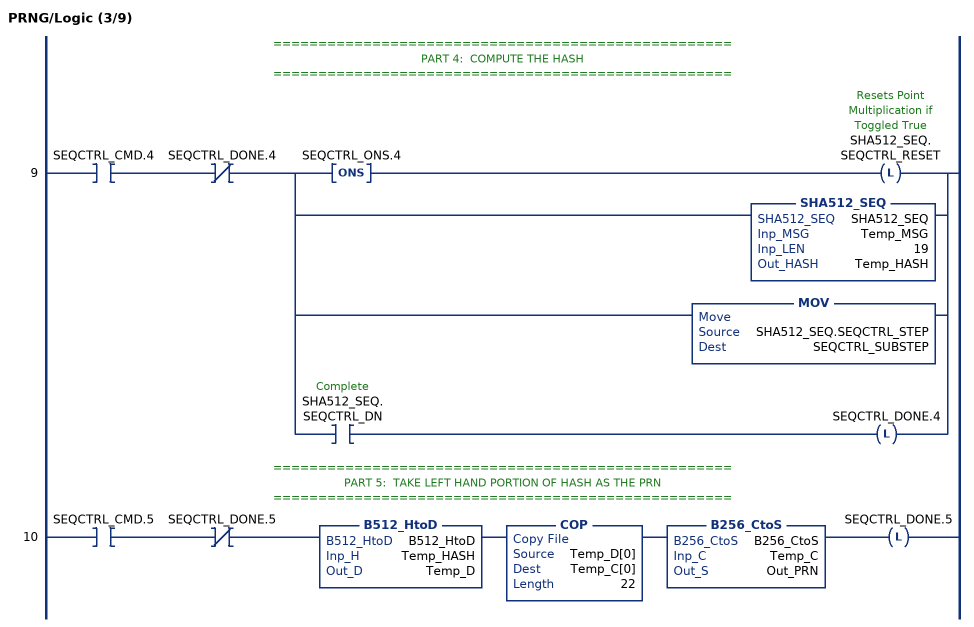
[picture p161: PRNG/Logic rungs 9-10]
   // ===================================================
   // PART 4:  COMPUTE THE HASH
   // ===================================================
   9: XIC(SEQCTRL_CMD.4)XIO(SEQCTRL_DONE.4)[ONS(SEQCTRL_ONS.4) OTL(SHA512_SEQ.SEQCTRL_RESET) ,SHA512_SEQ(SHA512_SEQ,Temp_MSG,19,Temp_HASH) ,MOV(SHA512_SEQ.SEQCTRL_STEP,SEQCTRL_SUBSTEP) ,XIC(SHA512_SEQ.SEQCTRL_DN) OTL(SEQCTRL_DONE.4) ];
   // ===================================================
   // PART 5:  TAKE LEFT HAND PORTION OF HASH AS THE PRN
   // ===================================================
   10: XIC(SEQCTRL_CMD.5)XIO(SEQCTRL_DONE.5)B512_HtoD(B512_HtoD,Temp_HASH,Temp_D)COP(Temp_D[0],Temp_C[0],22)B256_CtoS(B256_CtoS,Temp_C,Out_PRN)OTL(SEQCTRL_DONE.5);
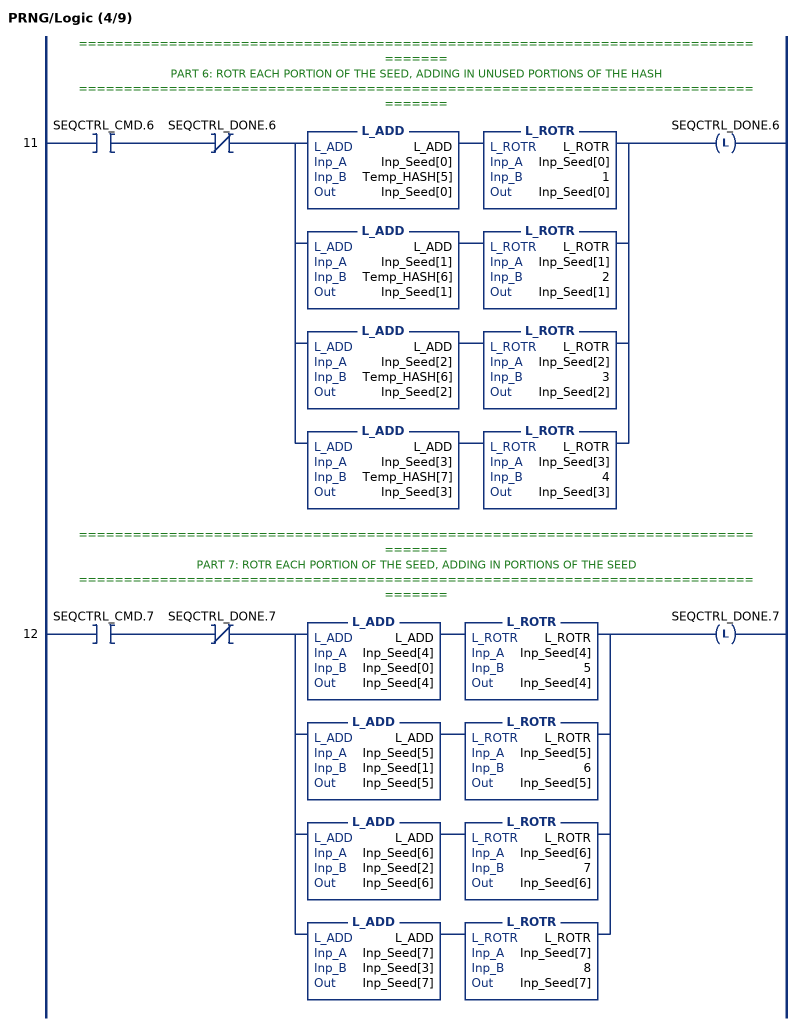
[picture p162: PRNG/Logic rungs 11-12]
   // ==================================================================================
   // PART 6: ROTR EACH PORTION OF THE SEED, ADDING IN UNUSED PORTIONS OF THE HASH
   // ==================================================================================
   11: XIC(SEQCTRL_CMD.6)XIO(SEQCTRL_DONE.6)[L_ADD(L_ADD,Inp_Seed[0],Temp_HASH[5],Inp_Seed[0]) L_ROTR(L_ROTR,Inp_Seed[0],1,Inp_Seed[0]) ,L_ADD(L_ADD,Inp_Seed[1],Temp_HASH[6],Inp_Seed[1]) L_ROTR(L_ROTR,Inp_Seed[1],2,Inp_Seed[1]) ,L_ADD(L_ADD,Inp_Seed[2],Temp_HASH[6],Inp_Seed[2]) L_ROTR(L_ROTR,Inp_Seed[2],3,Inp_Seed[2]) ,L_ADD(L_ADD,Inp_Seed[3],Temp_HASH[7],Inp_Seed[3]) L_ROTR(L_ROTR,Inp_Seed[3],4,Inp_Seed[3]) ]OTL(SEQCTRL_DONE.6);
   // ==================================================================================
   // PART 7: ROTR EACH PORTION OF THE SEED, ADDING IN PORTIONS OF THE SEED
   // ==================================================================================
   12: XIC(SEQCTRL_CMD.7)XIO(SEQCTRL_DONE.7)[L_ADD(L_ADD,Inp_Seed[4],Inp_Seed[0],Inp_Seed[4]) L_ROTR(L_ROTR,Inp_Seed[4],5,Inp_Seed[4]) ,L_ADD(L_ADD,Inp_Seed[5],Inp_Seed[1],Inp_Seed[5]) L_ROTR(L_ROTR,Inp_Seed[5],6,Inp_Seed[5]) ,L_ADD(L_ADD,Inp_Seed[6],Inp_Seed[2],Inp_Seed[6]) L_ROTR(L_ROTR,Inp_Seed[6],7,Inp_Seed[6]) ,L_ADD(L_ADD,Inp_Seed[7],Inp_Seed[3],Inp_Seed[7]) L_ROTR(L_ROTR,Inp_Seed[7],8,Inp_Seed[7]) ]OTL(SEQCTRL_DONE.7);
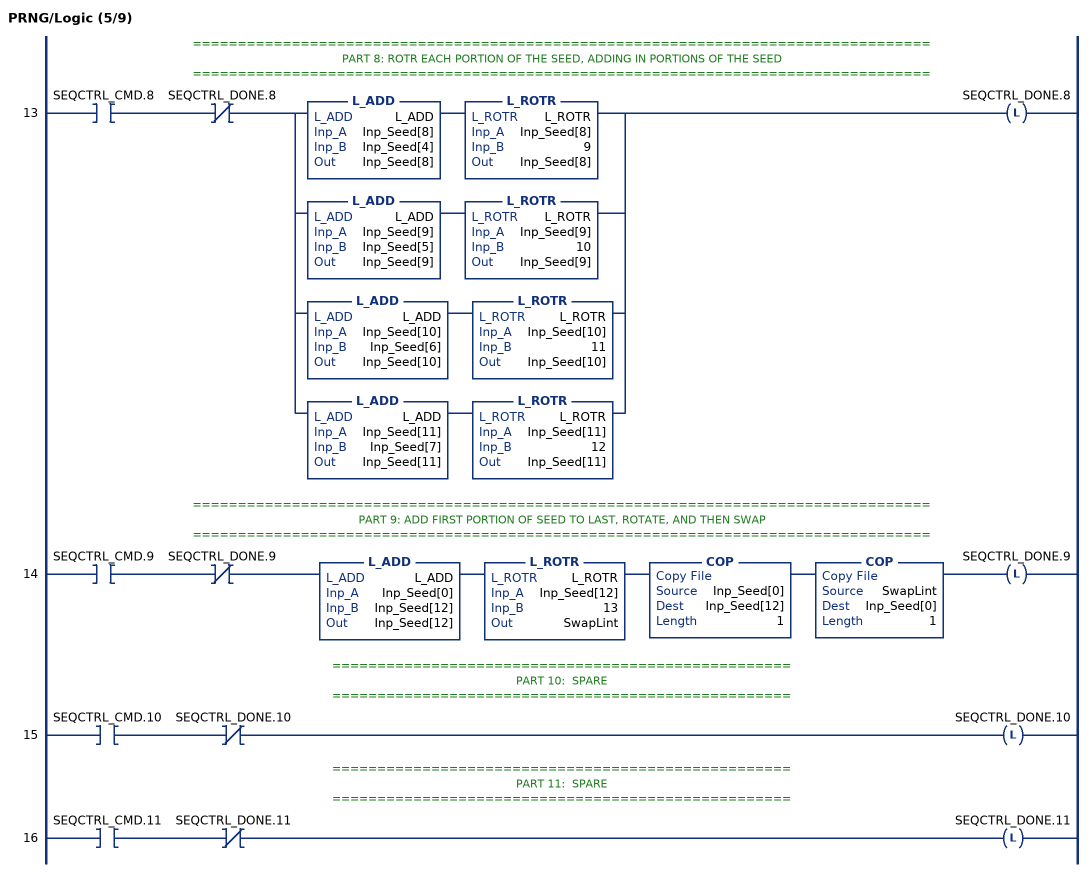
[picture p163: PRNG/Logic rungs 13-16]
   // ==================================================================================
   // PART 8: ROTR EACH PORTION OF THE SEED, ADDING IN PORTIONS OF THE SEED
   // ==================================================================================
   13: XIC(SEQCTRL_CMD.8)XIO(SEQCTRL_DONE.8)[L_ADD(L_ADD,Inp_Seed[8],Inp_Seed[4],Inp_Seed[8]) L_ROTR(L_ROTR,Inp_Seed[8],9,Inp_Seed[8]) ,L_ADD(L_ADD,Inp_Seed[9],Inp_Seed[5],Inp_Seed[9]) L_ROTR(L_ROTR,Inp_Seed[9],10,Inp_Seed[9]) ,L_ADD(L_ADD,Inp_Seed[10],Inp_Seed[6],Inp_Seed[10]) L_ROTR(L_ROTR,Inp_Seed[10],11,Inp_Seed[10]) ,L_ADD(L_ADD,Inp_Seed[11],Inp_Seed[7],Inp_Seed[11]) L_ROTR(L_ROTR,Inp_Seed[11],12,Inp_Seed[11]) ]OTL(SEQCTRL_DONE.8);
   // ==================================================================================
   // PART 9: ADD FIRST PORTION OF SEED TO LAST, ROTATE, AND THEN SWAP
   // ==================================================================================
   14: XIC(SEQCTRL_CMD.9)XIO(SEQCTRL_DONE.9)L_ADD(L_ADD,Inp_Seed[0],Inp_Seed[12],Inp_Seed[12])L_ROTR(L_ROTR,Inp_Seed[12],13,SwapLint)COP(Inp_Seed[0],Inp_Seed[12],1)COP(SwapLint,Inp_Seed[0],1)OTL(SEQCTRL_DONE.9);
   // ===================================================
   // PART 10:  SPARE
   // ===================================================
   15: XIC(SEQCTRL_CMD.10)XIO(SEQCTRL_DONE.10)OTL(SEQCTRL_DONE.10);
   // ===================================================
   // PART 11:  SPARE
   // ===================================================
   16: XIC(SEQCTRL_CMD.11)XIO(SEQCTRL_DONE.11)OTL(SEQCTRL_DONE.11);
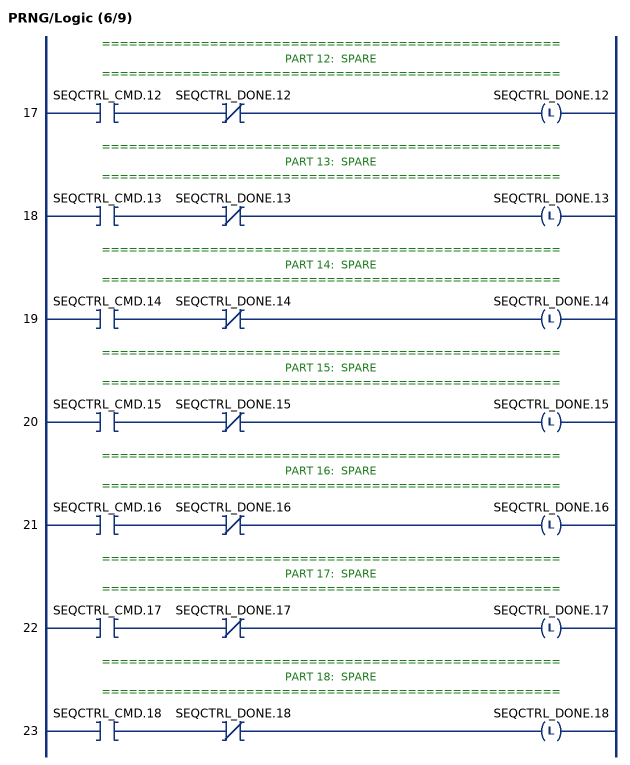
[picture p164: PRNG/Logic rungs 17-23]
   // ===================================================
   // PART 12:  SPARE
   // ===================================================
   17: XIC(SEQCTRL_CMD.12)XIO(SEQCTRL_DONE.12)OTL(SEQCTRL_DONE.12);
   // ===================================================
   // PART 13:  SPARE
   // ===================================================
   18: XIC(SEQCTRL_CMD.13)XIO(SEQCTRL_DONE.13)OTL(SEQCTRL_DONE.13);
   // ===================================================
   // PART 14:  SPARE
   // ===================================================
   19: XIC(SEQCTRL_CMD.14)XIO(SEQCTRL_DONE.14)OTL(SEQCTRL_DONE.14);
   // ===================================================
   // PART 15:  SPARE
   // ===================================================
   20: XIC(SEQCTRL_CMD.15)XIO(SEQCTRL_DONE.15)OTL(SEQCTRL_DONE.15);
   // ===================================================
   // PART 16:  SPARE
   // ===================================================
   21: XIC(SEQCTRL_CMD.16)XIO(SEQCTRL_DONE.16)OTL(SEQCTRL_DONE.16);
   // ===================================================
   // PART 17:  SPARE
   // ===================================================
   22: XIC(SEQCTRL_CMD.17)XIO(SEQCTRL_DONE.17)OTL(SEQCTRL_DONE.17);
   // ===================================================
   // PART 18:  SPARE
   // ===================================================
   23: XIC(SEQCTRL_CMD.18)XIO(SEQCTRL_DONE.18)OTL(SEQCTRL_DONE.18);
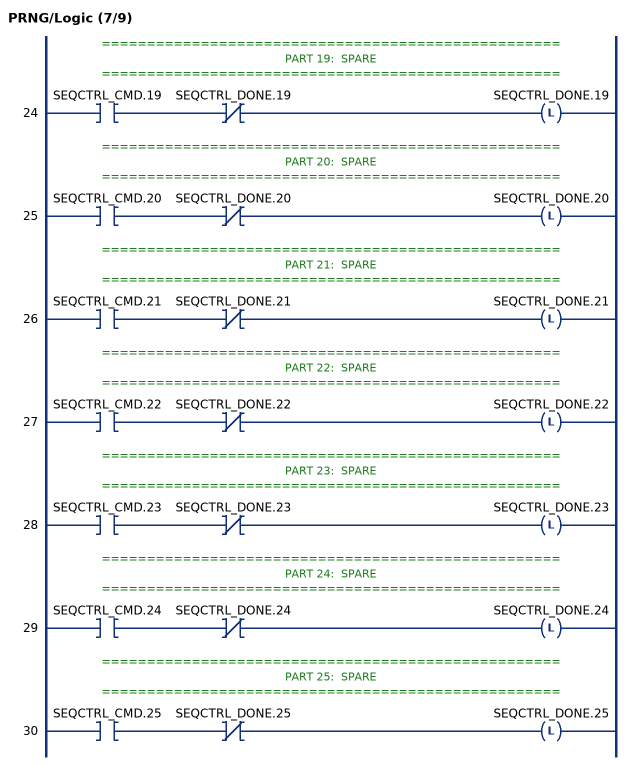
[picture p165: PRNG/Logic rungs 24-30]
   // ===================================================
   // PART 19:  SPARE
   // ===================================================
   24: XIC(SEQCTRL_CMD.19)XIO(SEQCTRL_DONE.19)OTL(SEQCTRL_DONE.19);
   // ===================================================
   // PART 20:  SPARE
   // ===================================================
   25: XIC(SEQCTRL_CMD.20)XIO(SEQCTRL_DONE.20)OTL(SEQCTRL_DONE.20);
   // ===================================================
   // PART 21:  SPARE
   // ===================================================
   26: XIC(SEQCTRL_CMD.21)XIO(SEQCTRL_DONE.21)OTL(SEQCTRL_DONE.21);
   // ===================================================
   // PART 22:  SPARE
   // ===================================================
   27: XIC(SEQCTRL_CMD.22)XIO(SEQCTRL_DONE.22)OTL(SEQCTRL_DONE.22);
   // ===================================================
   // PART 23:  SPARE
   // ===================================================
   28: XIC(SEQCTRL_CMD.23)XIO(SEQCTRL_DONE.23)OTL(SEQCTRL_DONE.23);
   // ===================================================
   // PART 24:  SPARE
   // ===================================================
   29: XIC(SEQCTRL_CMD.24)XIO(SEQCTRL_DONE.24)OTL(SEQCTRL_DONE.24);
   // ===================================================
   // PART 25:  SPARE
   // ===================================================
   30: XIC(SEQCTRL_CMD.25)XIO(SEQCTRL_DONE.25)OTL(SEQCTRL_DONE.25);
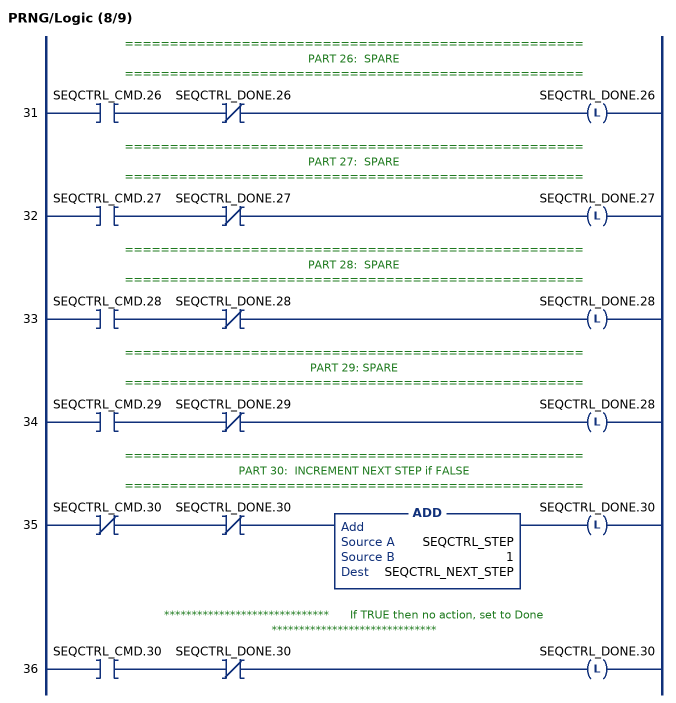
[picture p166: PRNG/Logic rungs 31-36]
   // ===================================================
   // PART 26:  SPARE
   // ===================================================
   31: XIC(SEQCTRL_CMD.26)XIO(SEQCTRL_DONE.26)OTL(SEQCTRL_DONE.26);
   // ===================================================
   // PART 27:  SPARE
   // ===================================================
   32: XIC(SEQCTRL_CMD.27)XIO(SEQCTRL_DONE.27)OTL(SEQCTRL_DONE.27);
   // ===================================================
   // PART 28:  SPARE
   // ===================================================
   33: XIC(SEQCTRL_CMD.28)XIO(SEQCTRL_DONE.28)OTL(SEQCTRL_DONE.28);
   // ===================================================
   // PART 29: SPARE
   // ===================================================
   34: XIC(SEQCTRL_CMD.29)XIO(SEQCTRL_DONE.29)OTL(SEQCTRL_DONE.28);
   // ===================================================
   // PART 30:  INCREMENT NEXT STEP if FALSE
   // ===================================================
   35: XIO(SEQCTRL_CMD.30)XIO(SEQCTRL_DONE.30)ADD(SEQCTRL_STEP,1,SEQCTRL_NEXT_STEP)OTL(SEQCTRL_DONE.30);
   // ******************************      If TRUE then no action, set to Done     ******************************
   36: XIC(SEQCTRL_CMD.30)XIO(SEQCTRL_DONE.30)OTL(SEQCTRL_DONE.30);
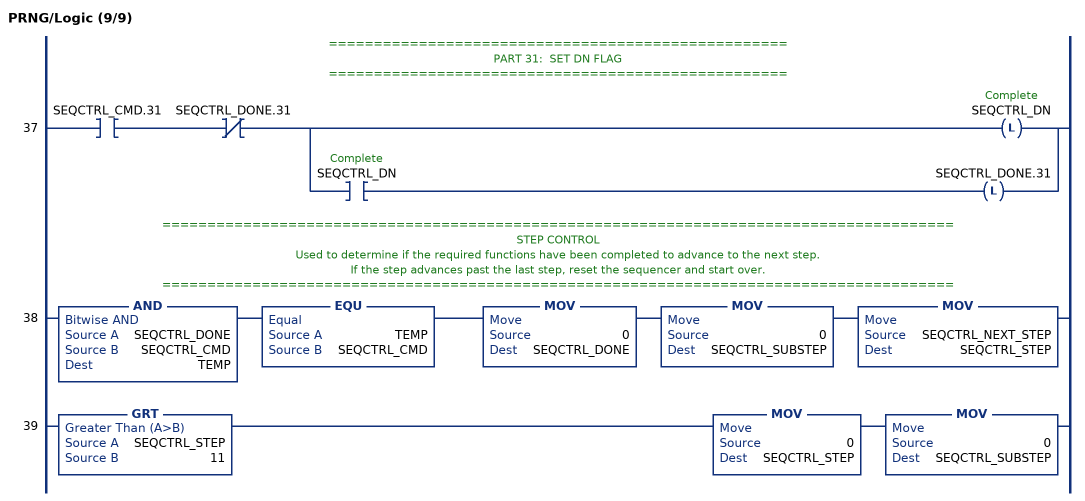
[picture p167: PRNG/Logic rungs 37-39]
   // ===================================================
   // PART 31:  SET DN FLAG
   // ===================================================
   37: XIC(SEQCTRL_CMD.31)XIO(SEQCTRL_DONE.31)[OTL(SEQCTRL_DN) ,XIC(SEQCTRL_DN) OTL(SEQCTRL_DONE.31) ];
   // ========================================================================================
   // STEP CONTROL
   // Used to determine if the required functions have been completed to advance to the next step.
   // If the step advances past the last step, reset the sequencer and start over.
   // ========================================================================================
   38: AND(SEQCTRL_DONE,SEQCTRL_CMD,TEMP)EQU(TEMP,SEQCTRL_CMD)MOV(0,SEQCTRL_DONE)MOV(0,SEQCTRL_SUBSTEP)MOV(SEQCTRL_NEXT_STEP,SEQCTRL_STEP);
   39: GRT(SEQCTRL_STEP,11)MOV(0,SEQCTRL_STEP)MOV(0,SEQCTRL_SUBSTEP);
END_ROUTINE
END_ADD_ON_INSTRUCTION
